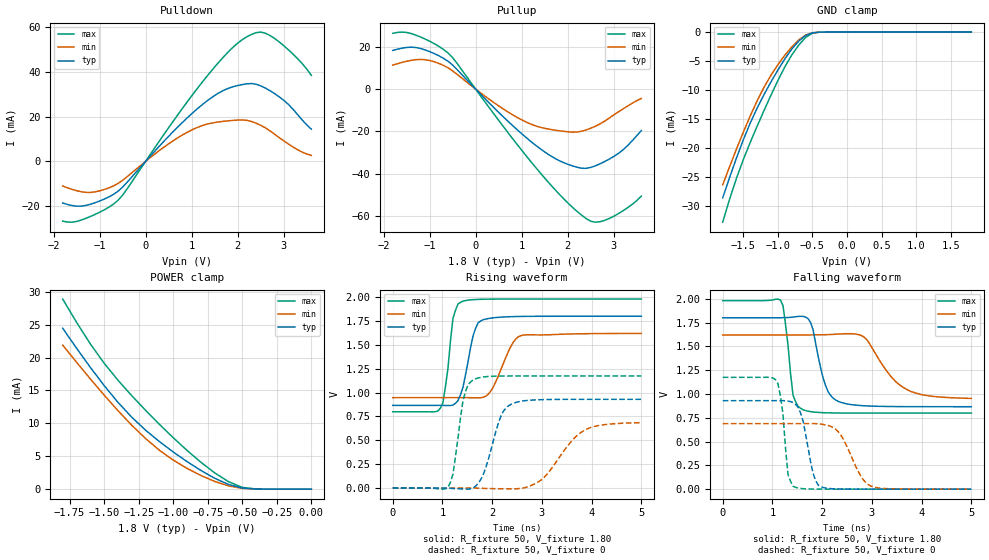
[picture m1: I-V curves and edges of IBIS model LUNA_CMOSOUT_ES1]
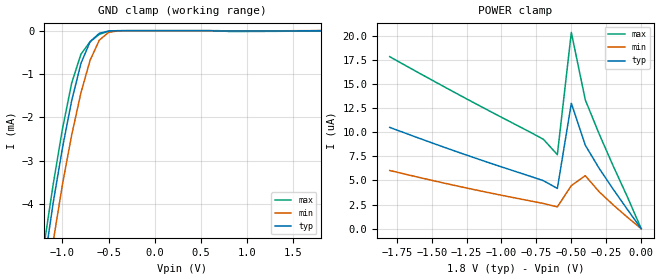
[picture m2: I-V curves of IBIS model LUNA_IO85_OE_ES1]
[IBIS Ver]   3.2
[Comment Char]   |_char
[File name]   sg-9101cx_18v_b.ibs
[File Rev]   1.0
[Date]   2020/01/21 10:45:03
[Source]
[Notes]
[Disclaimer]
This information is for modeling purposes only, and is not guaranteed.
Property of SEIKO EPSON Corp.,
unauthorized reproduction and/or distribution is strictly prohibited.
[Copyright]
Copyright 2020, SEIKO EPSON Corp.
[Component]   SG-9101CA
Si_location Pin
Timing_location Pin
[Manufacturer]   SEIKO EPSON Corp.
| 7050 PKG
| 7050 PKG
[Package]
R_pkg   224m   NA   NA
L_pkg   5.5n   NA   NA
C_pkg   0.144p   NA   NA
[Pin] signal_name   model_name
1   OE   LUNA_IO85_OE_ES1
2   VSS   GND
3   OUT   LUNA_CMOSOUT_ES1
4   VDD   POWER
[Component]   SG-9101CB
Si_location Pin
Timing_location Pin
[Manufacturer]   SEIKO EPSON Corp.
| 5032 PKG
| 5032 PKG
[Package]
R_pkg   200m   NA   NA
L_pkg   2.16n   NA   NA
C_pkg   1.23p   NA   NA
[Pin] signal_name   model_name
1   OE   LUNA_IO85_OE_ES1
2   VSS   GND
3   OUT   LUNA_CMOSOUT_ES1
4   VDD   POWER
[Component]   SG-9101CE
Si_location Pin
Timing_location Pin
[Manufacturer]   SEIKO EPSON Corp.
| 3225 PKG
| 3225 PKG
[Package]
R_pkg   177m   NA   NA
L_pkg   4.5n   NA   NA
C_pkg   0.64p   NA   NA
[Pin] signal_name   model_name
1   OE   LUNA_IO85_OE_ES1
2   VSS   GND
3   OUT   LUNA_CMOSOUT_ES1
4   VDD   POWER
[Component]   SG-9101CG
Si_location Pin
Timing_location Pin
[Manufacturer]   SEIKO EPSON Corp.
| 2520 PKG
| 2520 PKG
[Package]
R_pkg   238m   NA   NA
L_pkg   2.1n   NA   NA
C_pkg   0.38p   NA   NA
[Pin] signal_name   model_name
1   OE   LUNA_IO85_OE_ES1
2   VSS   GND
3   OUT   LUNA_CMOSOUT_ES1
4   VDD   POWER
| Models and submodels in the file (2): LUNA_CMOSOUT_ES1 (3-state), LUNA_IO85_OE_ES1 (Input)
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[Model]   LUNA_CMOSOUT_ES1
Model_type 3-state
Enable Active-High
Polarity Non-Inverting
Vmeas=0.90
C_comp   2.5p   2.0p   3.0p
[Temperature Range] 25   105   -40
[Voltage Range]   1.80   1.62   1.98
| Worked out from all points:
|   slope of the pulldown table from 0 to 0.27 V, typ, clamps not added: 43.9 ohm
|   slope of the pullup table from 0 to 0.27 V, typ, clamps not added: 44.8 ohm
|   GND clamp passes 1 mA (typ) near -0.64 V on its own axis
|   POWER clamp passes 1 mA (typ) near -0.63 V on its own axis
|   falling waveform, R_fixture 50, V_fixture 1.80: 20-80 % time 257ps typ, 580ps min, 144ps max; typ from 1.8 V to 0.866 V
|   falling waveform, R_fixture 50, V_fixture 0: 20-80 % time 210ps typ, 382ps min, 127ps max; typ from 0.929 V to 0 V
|   rising waveform, R_fixture 50, V_fixture 1.80: 20-80 % time 217ps typ, 334ps min, 152ps max; typ from 0.866 V to 1.8 V
|   rising waveform, R_fixture 50, V_fixture 0: 20-80 % time 317ps typ, 612ps min, 189ps max; typ from 0 V to 0.929 V
[Pullup]
-1.8V     18.24mA    11.3mA     26.32mA
-1.3V     19.62mA    13.85mA    25.49mA
-1V       17.7mA     13.49mA    22.61mA
-600mV    13.15mA    10.04mA    17.03mA
400mV     -8.857mA   -6.446mA   -11.85mA
1.1V      -22.96mA   -15.62mA   -31.6mA
1.8V      -33.66mA   -19.67mA   -49.3mA
2.4V      -37.49mA   -19.34mA   -61.21mA
2.6V      -36.32mA   -17.61mA   -62.94mA
2.8V      -34.33mA   -15.24mA   -62.1mA
3.2V      -28.77mA   -9.441mA   -57.57mA
3.6V      -19.68mA   -4.442mA   -50.62mA
[Pulldown]
-1.8V     -18.57mA   -10.98mA   -26.65mA
-1.5V     -19.96mA   -13.06mA   -26.8mA
-1.2V     -19.13mA   -13.84mA   -24.58mA
-600mV    -13.35mA   -9.866mA   -17.4mA
400mV     9.024mA    6.374mA    12.07mA
1V        21.23mA    14mA       29.2mA
1.6V      30.67mA    17.66mA    44.51mA
2.2V      34.62mA    18.33mA    55.63mA
2.5V      33.73mA    16.12mA    57.71mA
2.7V      31.58mA    13.67mA    56.21mA
3.2V      23.34mA    6.472mA    47.93mA
3.6V      14.38mA    2.699mA    38.41mA
[GND Clamp]
-1.8V     -28.67mA   -26.41mA   -32.88mA
-1.6V     -21.75mA   -20.22mA   -25.25mA
-1.5V     -18.58mA   -17.27mA   -22mA
-1.4V     -15.69mA   -14.46mA   -19.04mA
-1.2V     -10.77mA   -9.503mA   -13.52mA
-1.1V     -8.591mA   -7.44mA    -10.88mA
-900mV    -4.635mA   -4.001mA   -6.009mA
-700mV    -1.565mA   -1.365mA   -2.263mA
-600mV    -601.2uA   -521.6uA   -925.2uA
-500mV    -121.4uA   -116.4uA   -188.8uA
-400mV    -10.57uA   -14.63uA   -13.06uA
1.8V      99.8pA     105.8nA    71.35pA
[POWER Clamp]
-1.8V     24.46mA    21.89mA    28.9mA
-1.6V     18.52mA    16.76mA    22.08mA
-1.5V     15.75mA    14.3mA     19.15mA
-1.3V     10.93mA    9.714mA    14.21mA
-1.1V     7.236mA    5.92mA     9.861mA
-1V       5.655mA    4.424mA    7.824mA
-900mV    4.191mA    3.162mA    5.894mA
-700mV    1.665mA    1.179mA    2.483mA
-600mV    721.7uA    498.7uA    1.143mA
-500mV    167.2uA    126.9uA    275.1uA
-400mV    16.41uA    18.75uA    19.76uA
0V        99.8pA     596.4pA    86.97pA
[Falling Waveform]
R_fixture=50
V_fixture=1.80
V_fixture_min=1.62
V_fixture_max=1.98
0s        1.8V       1.62V      1.98V
1.162ns   1.8V       1.62V      1.985V
1.414ns   1.807V     1.62V      986.7mV
1.616ns   1.815V     1.62V      834mV
1.818ns   1.674V     1.62V      810.6mV
2.071ns   1.085V     1.622V     802.3mV
2.323ns   921.9mV    1.629V     799.9mV
2.879ns   874.7mV    1.581V     799mV
3.737ns   866.6mV    1.038V     799mV
5ns       866mV      952.9mV    799mV
[Falling Waveform]
R_fixture=50
V_fixture=0
V_fixture_min=0
V_fixture_max=0
0s        929.5mV    688.1mV    1.174V
1.061ns   929.4mV    688.1mV    1.15V
1.212ns   929.7mV    688.1mV    789.4mV
1.313ns   925.4mV    688.1mV    153.8mV
1.414ns   910mV      688.1mV    30.56mV
1.566ns   800.9mV    688mV      7.672mV
1.97ns    27.88mV    683.4mV    486.1uV
2.323ns   2.381mV    603.1mV    75.18uV
2.98ns    232.1uV    33.06mV    2.663uV
5ns       0V         114.1uV    0V
[Rising Waveform]
R_fixture=50
V_fixture=1.80
V_fixture_min=1.62
V_fixture_max=1.98
0s        866mV      947mV      799mV
959.6ps   866.2mV    947mV      838mV
1.061ns   865.2mV    947mV      1.062V
1.212ns   869mV      947mV      1.778V
1.414ns   1.057V     947.2mV    1.959V
1.616ns   1.595V     945.9mV    1.974V
1.818ns   1.764V     950.5mV    1.978V
2.02ns    1.783V     1.056V     1.98V
2.576ns   1.798V     1.596V     1.98V
5ns       1.8V       1.62V      1.98V
[Rising Waveform]
R_fixture=50
V_fixture=0
V_fixture_min=0
V_fixture_max=0
0s        0V         0V         0V
1.111ns   -978.3uV   2.379uV    5.98mV
1.212ns   -5.116mV   -5.883uV   146.2mV
1.414ns   -10.25mV   66.16uV    917.9mV
1.616ns   1.039mV    138.1uV    1.133V
2.172ns   747.2mV    -7.804mV   1.173V
2.374ns   875.9mV    -8.791mV   1.174V
2.98ns    925.9mV    81.76mV    1.174V
3.889ns   929.4mV    614.3mV    1.174V
5ns       929.5mV    685mV      1.174V
[Ramp]
R_load=50
dV/dt_r   5.577E-1/3.171E-10   4.110E-1/6.068E-10   7.045E-1/1.894E-10
dV/dt_f   5.604E-1/2.512E-10   4.003E-1/5.790E-10   7.086E-1/1.349E-10
|[End   LUNA_CMOSOUT_ES1
[Model]   LUNA_IO85_OE_ES1
Model_type Input
Enable Active-Low
Polarity Non-Inverting
Vinh=1.39
Vinl=0.48
C_comp   2.5p   2.0p   3.0p
[Temperature Range] 25   105   -40
[Voltage Range]   1.80   1.62   1.98
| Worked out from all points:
|   GND clamp passes 1 mA (typ) near -0.83 V on its own axis
[GND Clamp]
-1.8V     -17.06mA   -17.31mA   -17.53mA
-1.2V     -5.408mA   -6.351mA   -4.953mA
-1.1V     -3.959mA   -4.854mA   -3.533mA
-1V       -2.702mA   -3.543mA   -2.264mA
-900mV    -1.611mA   -2.406mA   -1.207mA
-800mV    -755.6uA   -1.435mA   -543.8uA
-700mV    -251.6uA   -679.9uA   -253.8uA
-600mV    -60.29uA   -218.4uA   -84.58uA
-500mV    -8.175uA   -39.66uA   -10.45uA
-400mV    -667.8nA   -4.047uA   -594nA
800mV     -9.61uA    -4.857uA   -17.73uA
1.8V      72.89pA    2.202uA    -5.276uA
[POWER Clamp]
-1.8V     10.5uA     6.032uA    17.83uA
-1.3V     7.877uA    4.371uA    13.84uA
-700mV    4.977uA    2.609uA    9.265uA
-600mV    4.168uA    2.258uA    7.669uA
-500mV    13uA       4.465uA    20.34uA
-400mV    8.645uA    5.49uA     13.35uA
-300mV    6.229uA    3.813uA    9.792uA
-200mV    4.08uA     2.459uA    6.49uA
-100mV    2.02uA     1.199uA    3.335uA
0V        72.85pA    181.7pA    73.98pA
